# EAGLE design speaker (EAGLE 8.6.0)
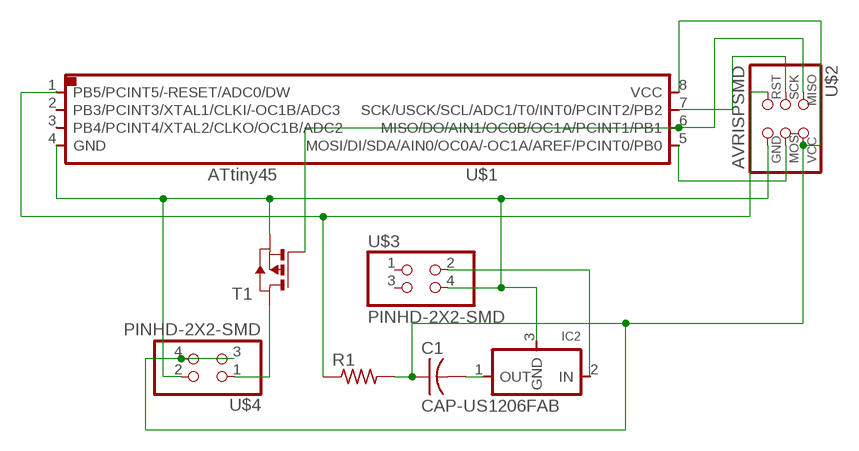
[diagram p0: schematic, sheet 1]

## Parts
C1  CAP-US1206FAB  [C1206FAB]
IC2  REGULATORSOT23  [SOT23]
R1  RES-US1206FAB  [R1206FAB]
T1  PMOSFETSOT23  [SOT-23]
U$1  ATTINY45SI  [SOIC8]
U$2  AVRISPSMD  [2X03SMD]
U$3  PINHD-2X2-SMD  [2X02SMD]
U$4  PINHD-2X2-SMD  [2X02SMD]

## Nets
N$1: U$1.5(MOSI/DI/SDA/AIN0/OC0A/-OC1A/AREF/PCINT0/PB0) U$2.4(MOSI)
N$2: U$1.7(SCK/USCK/SCL/ADC1/T0/INT0/PCINT2/PB2) U$2.3(SCK)
N$3: T1.3(G) U$1.6(MISO/DO/AIN1/OC0B/OC1A/PCINT1/PB1) U$2.1(MISO)
N$4: R1.1 U$1.1(PB5/PCINT5/-RESET/ADC0/DW) U$2.5(RST)
N$6: IC2.3(GND) T1.2(S) U$1.4(GND) U$2.6(GND) U$3.4 U$4.2
N$7: C1.2 IC2.1(OUT)
N$8: IC2.2(IN) U$3.2
N$9: T1.1(D) U$4.1
N$10: C1.1 R1.2 U$1.8(VCC) U$2.2(VCC) U$4.3 U$4.4
Unconnected: U$1.2(PB3/PCINT3/XTAL1/CLKI/-OC1B/ADC3) U$1.3(PB4/PCINT4/XTAL2/CLKO/OC1B/ADC2) U$3.1 U$3.3

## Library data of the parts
C1 = fab:CAP-US
IC2 = fab:REGULATOR
R1 = fab:RES-US: Resistor (US Symbol)
T1 = fab:PMOSFET: MOS FET
U$1 = fab:ATTINY45
U$2 = fab:AVRISP
U$3 U$4 = fab:PINHD-2X2-SMD

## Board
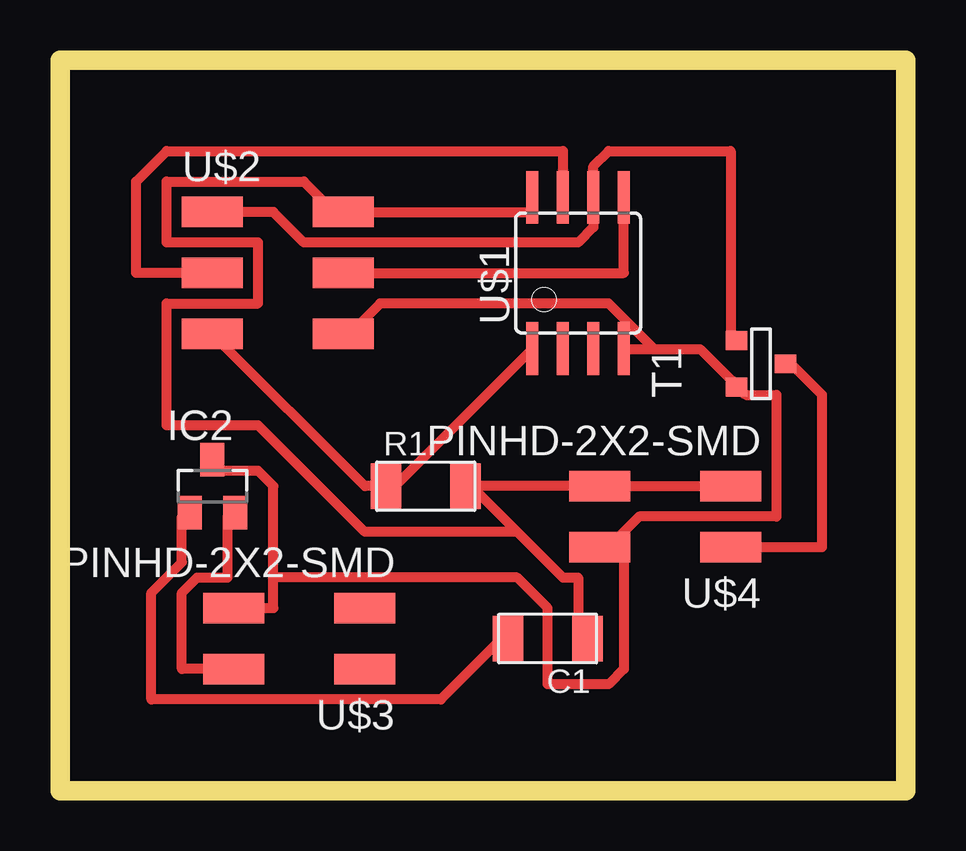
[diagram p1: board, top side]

Size 35.23 x 30.47 mm. Coordinates in mm from the lower left corner, seen from the top.
Outline: 0,0 35.23,0 35.23,30.47 0,30.47 0,0
Copper layers (1*16): Top 0.035mm / dielectric 1.5mm / Bottom 0.035mm
Design rules "default *": minimum track width 16mil, minimum drill 0.35mm, track to track 16mil, track to pad 16mil, pad to pad 16mil, via to via 16mil, smd to smd 16mil, copper to edge 40mil, drill to drill 16mil, minimum pad ring 10mil, minimum via ring 8mil, stop-mask expansion 4mil, vias tented up to drill 0mil, thermal gap 10mil

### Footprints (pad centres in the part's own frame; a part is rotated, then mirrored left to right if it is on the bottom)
C1206FAB = smd 1.27 x 1.905: 1 -1.651,0; 2 1.651,0
SOT23 = smd 1 x 1.4: 1 -0.95,-1.1; 2 0.95,-1.1; 3 0,1.1
R1206FAB = smd 1.27 x 1.905: 1 -1.651,0; 2 1.651,0
SOT-23 = smd 0.787 x 0.889: 1 0.025,-1.016; 2 -0.94,1.016; 3 0.991,1.016
SOIC8 = smd 0.5 x 2.2: 1 -1.905,-3.154; 2 -0.645,-3.154; 3 0.625,-3.154; 4 1.895,-3.154; 5 1.905,3.154; 6 0.635,3.154; 7 -0.635,3.154; 8 -1.905,3.154
2X03SMD = smd 2.54 x 1.27: 1 -2.54,2.54; 2 2.92,2.54; 3 -2.54,0; 4 2.92,0; 5 -2.54,-2.54; 6 2.92,-2.54
2X02SMD = smd 2.54 x 1.27: 1 -2.54,1.27; 2 2.92,1.27; 3 -2.54,-1.27; 4 2.92,-1.27

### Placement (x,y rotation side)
C1  20.32,6.35 180 top
IC2  6.35,12.7 0 top
R1  15.24,12.7 0 top
T1  29.21,17.78 90 top
U$1  21.59,21.59 0 top
U$2  8.89,21.59 0 top
U$3  10.16,6.35 180 top
U$4  25.4,11.43 180 top

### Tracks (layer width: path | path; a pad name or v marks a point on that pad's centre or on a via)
N$1
  Top 0.406: U$1.5 23.5,21.59 U$2.4
N$2
  Top 0.406: U$1.7 20.96,26.67 4.44,26.67 3.17,25.4 3.17,21.59 U$2.3
N$3
  Top 0.406: T1.3 27.94,19.05 27.94,26.67 22.86,26.67 22.22,26.04 U$1.6 22.22,23.49 21.59,22.86 10.16,22.86 8.89,24.13 U$2.1
N$4
  Top 0.406: U$1.1 19.68,18.41 13.97,12.7 R1.1 12.7,12.7 U$2.5
N$6
  Top 0.406: 8.89,8.89 8.89,7.62 U$3.4 | 8.89,8.89 8.89,12.7 8.25,13.34 6.35,13.34 IC2.3 | 24.76,18.41 23.5,18.41 U$1.4 | 24.76,18.41 26.67,18.41 27.94,17.15 T1.2 28.57,16.51 29.84,16.51 29.84,11.43 24.13,11.43 22.86,10.16 | 24.76,18.41 22.86,20.32 13.33,20.32 12.07,19.05 U$2.6 | 8.89,8.89 19.05,8.89 20.32,7.62 20.32,4.45 22.86,4.45 23.5,5.08 23.5,10.16 22.86,10.16 | 22.86,10.16 U$4.2
N$7
  Top 0.406: IC2.1 5.08,11.43 5.08,9.52 3.81,8.25 3.81,3.81 15.87,3.81 18.41,6.35 C1.2
N$8
  Top 0.406: U$3.2 5.08,5.08 5.08,8.25 5.71,8.89 6.98,8.89 6.98,11.43 IC2.2
N$9
  Top 0.406: U$4.1 31.75,10.16 31.75,16.51 30.48,17.78 T1.1
N$10
  Top 0.406: U$1.8 19.68,24.13 U$2.2 11.43,24.13 10.16,25.4 4.44,25.4 4.44,22.86 8.25,22.86 8.25,20.32 4.44,20.32 4.44,15.24 8.25,15.24 12.7,10.8 19.05,10.8 | 17.14,12.7 U$4.4 U$4.3 | 17.14,12.7 19.05,10.8 | 19.05,10.8 20.96,8.89 21.59,8.89 21.59,6.35 C1.1 | 17.14,12.7 R1.2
